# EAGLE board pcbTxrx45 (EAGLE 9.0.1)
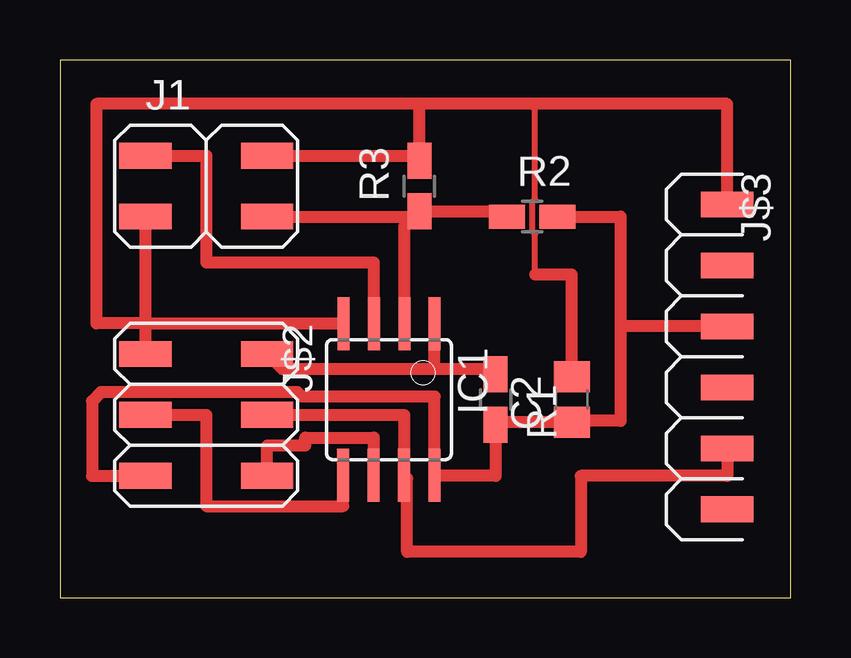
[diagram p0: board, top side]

Size 30.46 x 22.4 mm. Coordinates in mm from the lower left corner, seen from the top.
Outline: 0,0 30.46,0 30.46,22.4 0,22.4 0,0
Copper layers (1*16): Top 0.035mm / dielectric 1.5mm / Bottom 0.035mm
Design rules "default": minimum track width 6mil, minimum drill 0.35mm, track to track 6mil, track to pad 6mil, pad to pad 6mil, via to via 6mil, smd to smd 6mil, copper to edge 40mil, drill to drill 6mil, minimum pad ring 10mil, minimum via ring 8mil, stop-mask expansion 4mil, vias tented up to drill 0mil, thermal gap 10mil
Net classes: 0 default: width 0.254 mm

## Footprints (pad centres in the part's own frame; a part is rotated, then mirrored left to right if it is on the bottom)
C0805 = smd 1.3 x 1.5: 1 -0.95,0; 2 0.95,0
SOIC8 = smd 0.5 x 2.2: 1 -1.905,-3.154; 2 -0.645,-3.154; 3 0.625,-3.154; 4 1.895,-3.154; 5 1.905,3.154; 6 0.635,3.154; 7 -0.635,3.154; 8 -1.905,3.154
2X02 = smd 2.184 x 1.067: P$1 -2.54,-1.27; P$2 -2.54,1.27; P$3 2.54,-1.27; P$4 2.54,1.27
2X03 = smd 1.067 x 2.184: P$1 -2.54,-2.54; P$2 -2.54,2.54; P$3 0,-2.54; P$4 0,2.54; P$5 2.54,-2.54; P$6 2.54,2.54
1X06 = smd 1.067 x 2.184: P$1 -6.35,1.27; P$2 -3.81,1.27; P$3 -1.27,1.27; P$4 1.27,1.27; P$5 3.81,1.27; P$6 6.35,1.27
R0805W = smd 1.5 x 1: 1 -1.052,0; 2 1.052,0

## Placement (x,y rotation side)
C2  1uF  [C0805]  21.34,8.26 90 top
IC1  TINY45S  [SOIC8]  13.72,8.26 180 top
J1  PINSHD-2x2  [2X02]  6.1,17.14 0 top
J$2  PINSHD-2X3  [2X03]  6.1,7.62 270 top
J$3  PINSHD-1X6S  [1X06]  26.54,10.03 270 top
R1  10k  [R0805W]  18.16,8.26 270 top
R2  1M  [R0805W]  19.68,15.88 0 top
R3  1M  [R0805W]  14.99,17.14 90 top

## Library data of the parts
C2 R1-R3 = resistor
IC1 = atmel_mcu
J1 J$2 J$3 = pinhead_smd

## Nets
+3V3: C2.1 IC1.8 J$2.P$5 J$3.P$3 R1.2 R2.2
GND: C2.2 IC1.4 J1.P$1 J1.P$4 J$2.P$1 J$3.P$1 R3.2
MISO: IC1.6 J$2.P$6
MOSI: IC1.5 J$2.P$3
PRX: IC1.2 J1.P$3 R2.1 R3.1
PTX: IC1.3 J1.P$2
RESET: IC1.1 J$2.P$2 R1.1
SCK-RX: IC1.7 J$2.P$4 J$3.P$5

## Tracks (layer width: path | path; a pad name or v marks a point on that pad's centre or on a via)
+3V3
  Top 0.508: J$2.P$5 1.33,5.08 1.33,8.19 1.7,8.56 9.9,8.56 10.07,8.38 15.62,8.38 IC1.8 15.64,5.08 18.16,5.08 R1.2 18.26,7.31 C2.1 21.4,7.37 23.37,7.37 23.37,11.3 | R2.2 23.37,15.88 23.37,11.3 | J$3.P$3 23.37,11.3
GND
  Top 0.254: 19.68,20.57 19.81,20.45 19.81,16.59 19.71,16.49 19.71,15.26 19.81,15.15 19.81,13.46
  Top 0.508: J1.P$4 14.77,18.41 R3.2 14.99,20.57 | J1.P$1 3.56,11.43 | 3.56,11.43 J$2.P$1 | IC1.4 3.58,11.41 3.56,11.43 | J$3.P$1 27.81,20.57 19.68,20.57 14.99,20.57 | 14.99,20.57 1.52,20.57 1.52,11.43 3.56,11.43 | C2.2 21.34,13.46 19.81,13.46
MISO
  Top 0.508: J$2.P$6 8.64,6.35 10.22,6.35 10.22,6.67 13.08,6.67 IC1.6
MOSI
  Top 0.508: J$2.P$3 6.1,7.62 6.1,3.81 11.81,3.81 IC1.5
PRX
  Top 0.508: J1.P$3 14.77,15.88 | 14.77,15.88 R3.1 18.41,16.09 R2.1 | IC1.2 14.36,15.47 14.77,15.88
PTX
  Top 0.508: J1.P$2 6.1,18.41 6.1,13.97 13.08,13.97 13.08,11.42 IC1.3
RESET
  Top 0.508: R1.1 17.94,9.53 15.62,9.53 | 15.62,9.53 IC1.1 | 15.62,9.53 9.27,9.53 J$2.P$2
SCK-RX
  Top 0.508: J$2.P$4 14.35,7.62 IC1.7 14.48,4.97 14.48,1.91 21.72,1.91 21.72,5.08 27.81,5.08 J$3.P$5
